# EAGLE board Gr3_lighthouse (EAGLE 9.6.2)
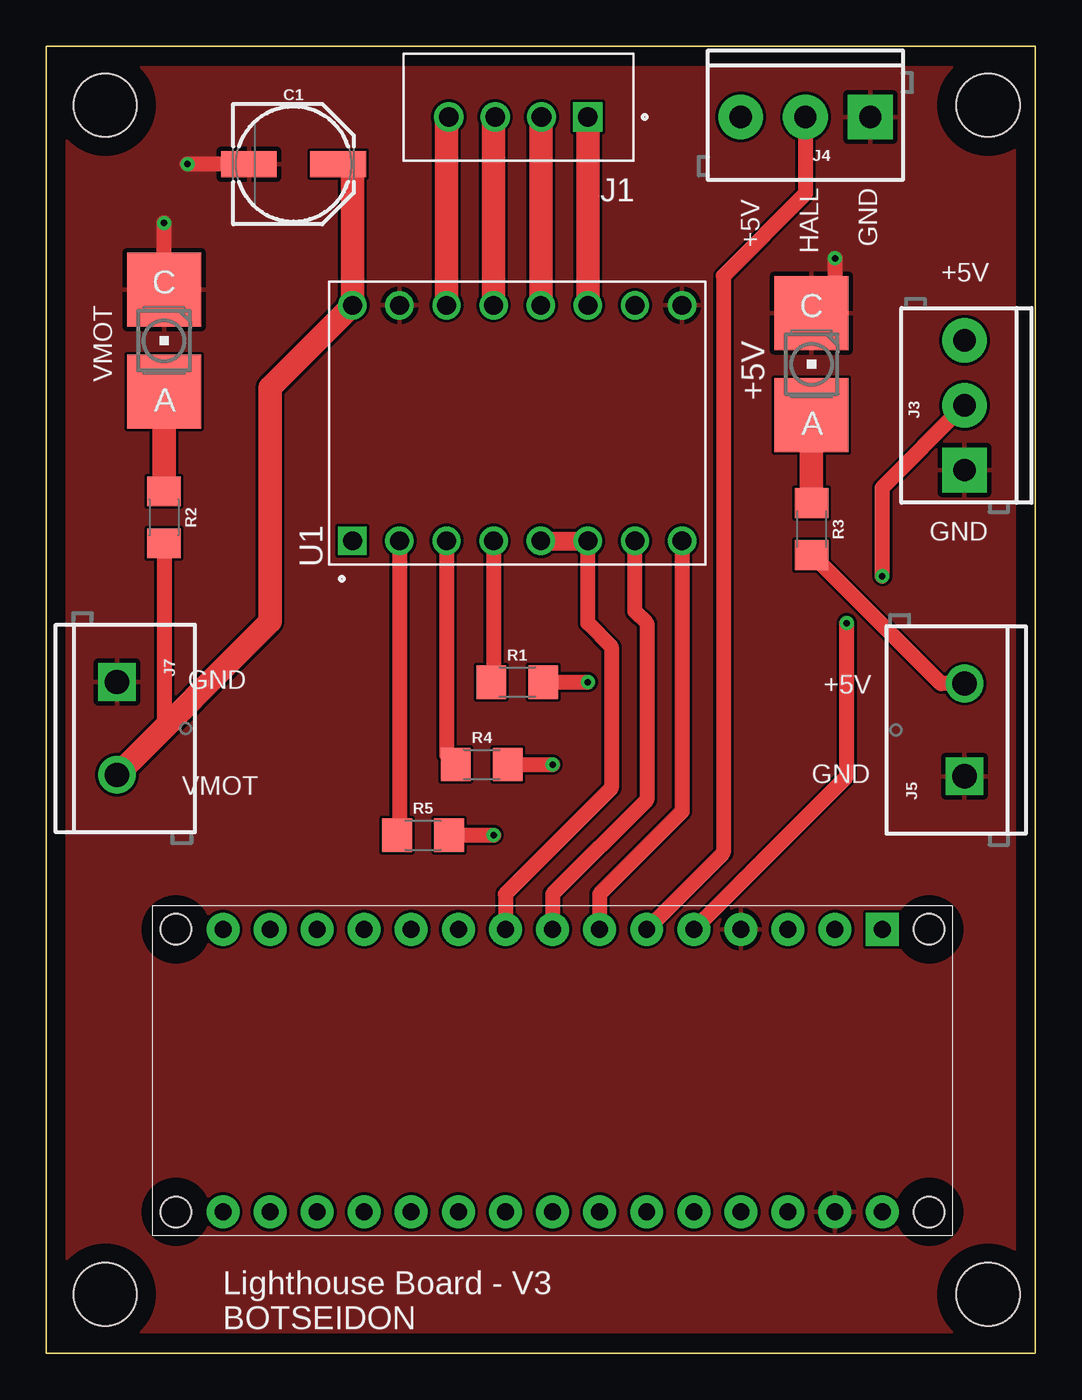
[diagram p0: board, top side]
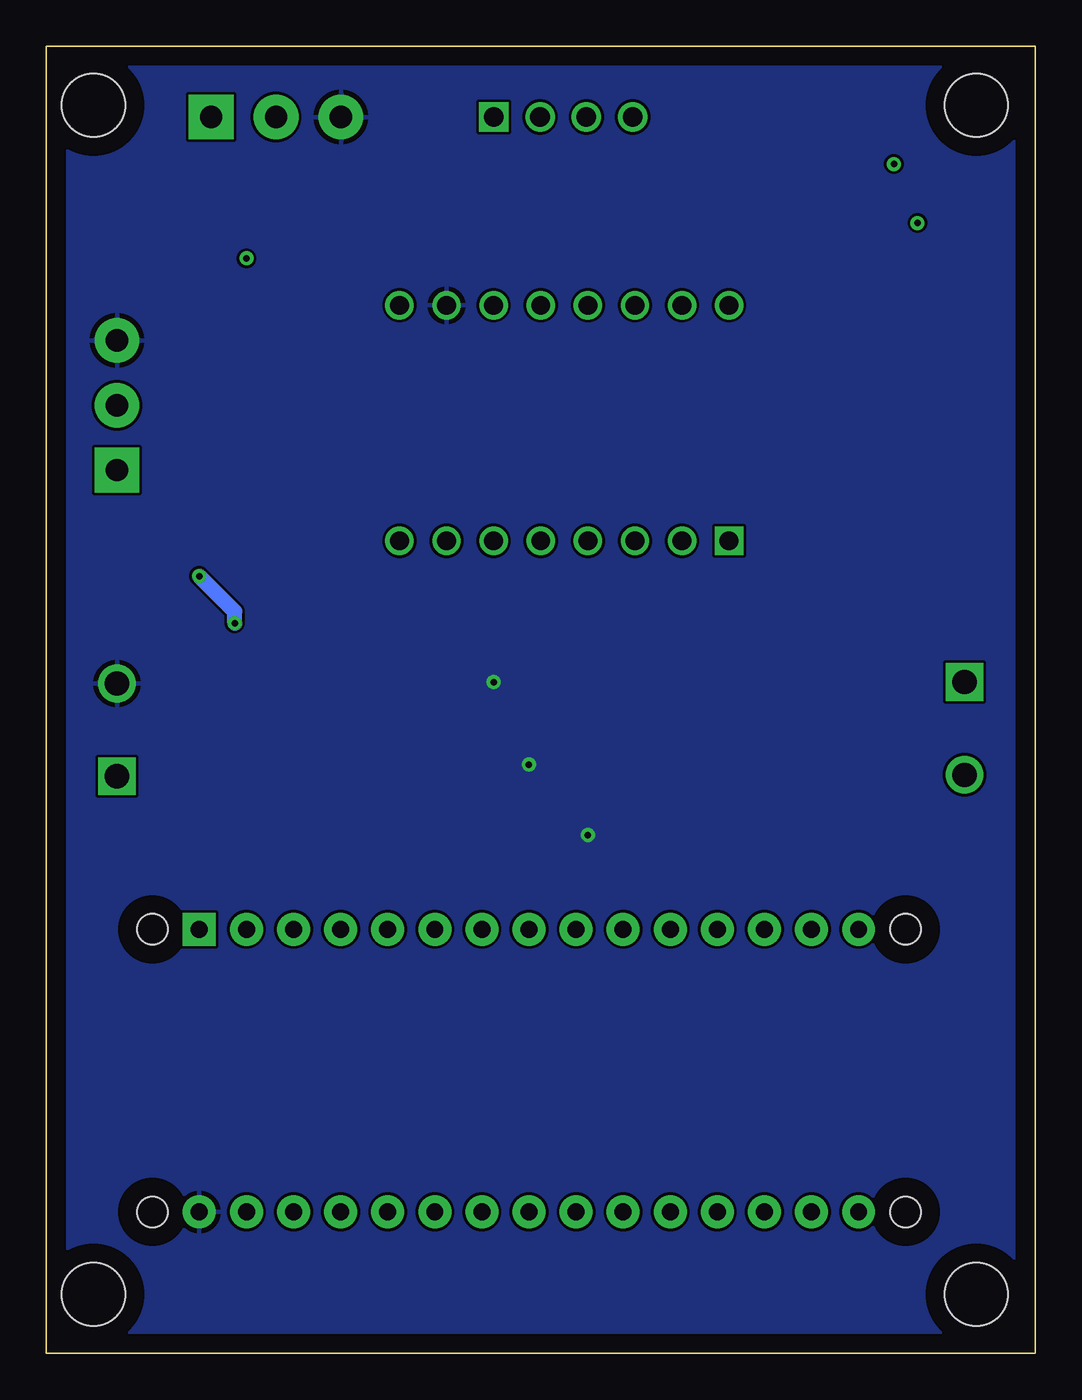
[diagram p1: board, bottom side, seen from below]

Size 53.34 x 70.48 mm. Coordinates in mm from the lower left corner, seen from the top.
Outline: 0,0 0,70.48 53.34,70.48 53.34,0 0,0
Copper layers (1*16): Top 0.035mm / dielectric 1.5mm / Bottom 0.035mm
Design rules "default": minimum track width 6mil, minimum drill 0.35mm, track to track 6mil, track to pad 6mil, pad to pad 6mil, via to via 6mil, smd to smd 6mil, copper to edge 40mil, drill to drill 6mil, minimum pad ring 10mil, minimum via ring 8mil, stop-mask expansion 4mil, vias tented up to drill 0mil, thermal gap 10mil
Holes 3.43 mm at 3.17,3.17 50.8,3.17 3.17,67.31 50.8,67.31

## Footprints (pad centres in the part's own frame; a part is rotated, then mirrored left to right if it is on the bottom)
P-LCC-2 = smd 4 x 4: A 0,2.75; C 0,-2.75
PANASONIC_D = smd 3 x 1.4: + 2.4,0; - -2.4,0
JST_B4B-XH-A(LF)(SN) = drill 1.06 square: 1 0,0 | drill 1.06: 2 2.5,0; 3 5,0; 4 7.5,0
SCREWTERMINAL-3.5MM-3 = drill 1.2 pad 2.413 square: 1 0,0 | drill 1.2 pad 2.413: 2 3.5,0; 3 7,0
SCREWTERMINAL-5MM-2 = drill 1.3 pad 2.032 square: 1 0,0 | drill 1.3 pad 2.032: 2 5,0
ARDUINO_NANO2 = drill 0.914 pad 1.778 square: J1.1 -7.62,17.78 | drill 0.914 pad 1.778: J1.2 -7.62,15.24; J1.3 -7.62,12.7; J1.4 -7.62,10.16; J1.5 -7.62,7.62; J1.6 -7.62,5.08; J1.7 -7.62,2.54; J1.8 -7.62,0; J1.9 -7.62,-2.54; J1.10 -7.62,-5.08; J1.11 -7.62,-7.62; J1.12 -7.62,-10.16; J1.13 -7.62,-12.7; J1.14 -7.62,-15.24; J1.15 -7.62,-17.78; J2.1 7.62,17.78; J2.2 7.62,15.24; J2.3 7.62,12.7; J2.4 7.62,10.16; J2.5 7.62,7.62; J2.6 7.62,5.08; J2.7 7.62,2.54; J2.8 7.62,0; J2.9 7.62,-2.54; J2.10 7.62,-5.08; J2.11 7.62,-7.62; J2.12 7.62,-10.16; J2.13 7.62,-12.7; J2.14 7.62,-15.24; J2.15 7.62,-17.78 | hole 1.651: -7.62,-20.32; 7.62,-20.32; 7.62,20.32; -7.62,20.32
1206 = smd 1.6 x 1.8: 1 -1.4,0; 2 1.4,0
MODULE_A4988_STEPPER_MOTOR_DRIVER_CARRIER = drill 1.02 square: 1 -6.35,8.89 | drill 1.02: 2 -6.35,6.35; 3 -6.35,3.81; 4 -6.35,1.27; 5 -6.35,-1.27; 6 -6.35,-3.81; 7 -6.35,-6.35; 8 -6.35,-8.89; 9 6.35,-8.89; 10 6.35,-6.35; 11 6.35,-3.81; 12 6.35,-1.27; 13 6.35,1.27; 14 6.35,3.81; 15 6.35,6.35; 16 6.35,8.89

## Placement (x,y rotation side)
+5V  [P-LCC-2]  41.27,53.34 180 top
C1  100uF  [PANASONIC_D]  13.34,64.14 0 top
J1  B4B-XH-A(LF)(SN)  [JST_B4B-XH-A(LF)(SN)]  29.21,66.67 180 top
J3  [SCREWTERMINAL-3.5MM-3]  49.53,47.62 90 top
J4  [SCREWTERMINAL-3.5MM-3]  44.45,66.67 180 top
J5  [SCREWTERMINAL-5MM-2]  49.53,31.11 90 top
J7  [SCREWTERMINAL-5MM-2]  3.81,36.2 270 top
MODUL1  ARDUINO_NANO2  [ARDUINO_NANO2]  27.3,15.24 270 top
R1  0  [1206]  25.4,36.2 0 top
R2  2.2k  [1206]  6.35,45.09 270 top
R3  1k  [1206]  41.27,44.45 270 top
R4  0  [1206]  23.5,31.75 0 top
R5  0  [1206]  20.32,27.94 0 top
U1  A4988_STEPPER_MOTOR_DRIVER_CARRIER  [MODULE_A4988_STEPPER_MOTOR_DRIVER_CARRIER]  25.4,50.16 90 top
VMOT  [P-LCC-2]  6.35,54.61 180 top

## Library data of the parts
+5V VMOT = adafruit
C1 = SparkFun-Capacitors; PROD_ID: CAP-12547
J1 = B4B-XH-A_LF__SN_; AVAILABILITY: Warning; DESCRIPTION: Connector Header Through Hole 4 position 0.098 (2.50mm); MF: JST Sales; MP: B4B-XH-A(LF)(SN); PACKAGE: None; PRICE: None; PURCHASE-URL: https://pricing.snapeda.com/search/part/B4B-XH-A(LF)(SN)/?ref=eda
J3 J4 = SparkFun-Connectors; PROD_ID: CONN-08288; SF_ID: PRT-08235
J5 J7 = SparkFun-Connectors; SF_SKU: PRT-08432
MODUL1 = arduino; ANZAHL: 2; MODUL: TRUE; STECKX0: -76200; STECKX1: 76200; STECKY0: 177800; STECKY1: 177800
R1-R5 = SparkFun-Resistors
U1 = A4988_STEPPER_MOTOR_DRIVER_CARRIER; AVAILABILITY: Unavailable; DESCRIPTION: Stepper Motor Driver; MF: Pololu; MP: A4988 STEPPER MOTOR DRIVER CARRIER; PACKAGE: None; PRICE: None

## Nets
3V3: MODUL1.J2.14
5V: J3.3 J4.3 J5.2 MODUL1.J2.1 R1.2 R3.2 R4.2 R5.2 U1.10
12V: C1.+ J7.2 R2.2 U1.16
+5V: MODUL1.J2.4
AREF: MODUL1.J2.13
DIR: MODUL1.J1.7 U1.8
GND: +5V.C C1.- J3.1 J4.1 J5.1 J7.1 MODUL1.J1.4 MODUL1.J2.2 U1.9 U1.15 VMOT.C
HALL: J4.2 MODUL1.J1.6
LEDS: J3.2 MODUL1.J1.5
N$1: +5V.A R3.1
N$3: R2.1 VMOT.A
N$7: J1.4 U1.14
N$8: J1.3 U1.13
N$9: J1.1 U1.11
N$10: J1.2 U1.12
N$11: R1.1 U1.4
N$12: R4.1 U1.3
N$13: R5.1 U1.2
SLEEP: MODUL1.J1.9 U1.5 U1.6
STEP: MODUL1.J1.8 U1.7

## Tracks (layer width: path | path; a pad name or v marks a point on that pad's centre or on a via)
5V  (via drill 0.35)
  Top 0.813: R5.2 v24.13,27.94 | R4.2 v27.3,31.75 | R1.2 v29.21,36.2 | J5.2 48.26,36.12 41.33,43.05 R3.2
  pour Bottom: 0,70.48 53.34,70.48 53.34,0 0,0
12V
  Top 0.813: R2.2 6.35,33.73 J7.2
  Top 1.27: C1.+ 16.51,64.14 U1.16 12.06,52.07 12.06,39.45 J7.2
DIR
  Top 0.813: MODUL1.J1.7 29.84,24.77 34.29,29.21 U1.8
GND  (via drill 0.35)
  Top 0.813: C1.- v7.62,64.14 | +5V.C 41.27,56.52 41.91,57.15 42.55,57.78 v42.55,59.05 | VMOT.C v6.35,60.96
  pour Top: 0,70.48 53.34,70.48 53.34,0 0,0
HALL
  Top 0.813: MODUL1.J1.6 36.51,26.99 36.51,58.1 40.95,62.54 J4.2
LEDS  (via drill 0.35)
  Top 0.813: v43.18,39.37 43.18,31.11 MODUL1.J1.5 | v45.09,41.91 45.09,46.68 J3.2
  Bottom 0.813: v45.09,41.91 43.18,40.01 v43.18,39.37
N$1
  Top 1.27: +5V.A R3.1
N$3
  Top 1.27: R2.1 VMOT.A
N$7
  Top 1.27: U1.14 21.59,66.56 J1.4
N$8
  Top 1.27: U1.13 24.13,66.59 J1.3
N$9
  Top 1.27: U1.11 J1.1
N$10
  Top 1.27: U1.12 26.67,66.64 J1.2
N$11
  Top 0.813: U1.4 24.13,36.33 R1.1
N$12
  Top 0.813: U1.3 21.59,32.26 R4.1
N$13
  Top 0.813: U1.2 19.05,28.07 R5.1
SLEEP
  Top 0.813: U1.6 29.21,39.37 30.48,38.1 30.48,30.48 24.77,24.77 MODUL1.J1.9
  Top 1.016: U1.5 U1.6
STEP
  Top 0.813: U1.7 31.75,40.01 32.38,39.37 32.38,29.84 27.3,24.77 MODUL1.J1.8

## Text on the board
tNames: HALL | GND | +5V | +5V | GND | GND | +5V | GND | VMOT | Lighthouse Board - V3 / BOTSEIDON

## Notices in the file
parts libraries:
SparkFun-Capacitors: Licensing: Creative Commons ShareAlike 4.0 International - https://creativecommons.org/licenses/by-sa/4.0
